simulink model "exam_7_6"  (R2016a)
settings: Solver=VariableStepAuto  StartTime=0.0  StopTime=10.0  RelTol=1e-3

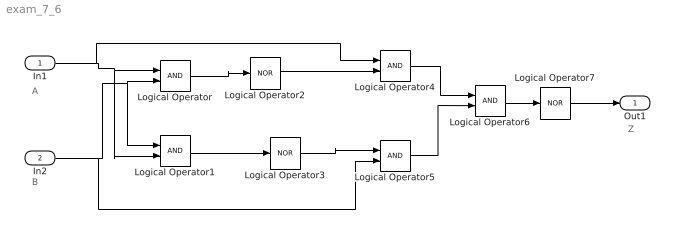
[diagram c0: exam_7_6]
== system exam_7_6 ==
  note: Z
  note: B
  note: A
  In1 : Inport
  In2 : Inport  Port=2
  Logical Operator{,1,4..6} (5 alike) : Logic  AllPortsSameDT=off  OutDataTypeStr=boolean
  Logical Operator2 : Logic  Operator=NOR  Inputs=1  AllPortsSameDT=off  OutDataTypeStr=boolean
  Logical Operator3 : Logic  Operator=NOR  Inputs=1  AllPortsSameDT=off  OutDataTypeStr=boolean
  Logical Operator7 : Logic  Operator=NOR  Inputs=1  AllPortsSameDT=off  OutDataTypeStr=boolean
  Out1 : Outport
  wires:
  In1/1 -> Logical Operator4/1, Logical Operator1/2, Logical Operator/1
  In2/1 -> Logical Operator5/2, Logical Operator1/1, Logical Operator/2
  Logical Operator/1 -> Logical Operator2/1
  Logical Operator2/1 -> Logical Operator4/2
  Logical Operator1/1 -> Logical Operator3/1
  Logical Operator3/1 -> Logical Operator5/1
  Logical Operator4/1 -> Logical Operator6/1
  Logical Operator5/1 -> Logical Operator6/2
  Logical Operator6/1 -> Logical Operator7/1
  Logical Operator7/1 -> Out1/1
